FUNCTION_BLOCK FB95
TITLE =Get Operation Mode
//*****************************************************************************
//* maxon motor ag
//* R&D
//* all rights reserved
//*****************************************************************************
//* Summary:  Read operation mode
//*
//* Remarks:
//*
//* Created under: STEP7 REV5.2+SP1
//*****************************************************************************
//* History:
//* 19.05.2004 | INA   first release
//*
//*
//*****************************************************************************
//

AUTHOR:INA
FAMILY:StateMac
NAME:GetOpMod
VERSION:00.01


VAR_INPUT

Read : BOOL //A rising edge start the command

  NodeID : BYTE //Adress of the maxon device

END_VAR
VAR_OUTPUT
  Done : BOOL //Data valid flag is TRUE if data were available

  Err : BOOL //Error flag is TRUE if an Error has occured, see ErrNo for more details

  ErrNo : DINT //Contains detailed error information

  Mode : BYTE //Operation Mode

END_VAR
VAR
  xEdgeMerker : BOOL //Edge Merker

  xEdgeFlag : BOOL //Edge Flag

  xStep : INT
END_VAR

BEGIN

NETWORK
TITLE = Activate the service function
//

// SDO Read "Get Operation Mode"

       U    #Read
       FP   #xEdgeFlag                   // recognize a positiv edge of the Read signal
       =    #xEdgeMerker                 // and set the xEdgeMerker for one cycle to true

       L    #xStep
       L    0
       ==I
       U    #xEdgeMerker
       SPB  nstp                         // iStep = 1 -> fnc1

       L    #xStep                       // jump list
       SPL  List
       SPA  rdef
       SPA  fnc1
       SPA  fncE
List  :SPA  rdef

rdef  :NOP  0
       R    #Done                        // reset Done
       R    #Err                         // reset Error
       L    0
       T    #xStep                       // iStep = 0
       SPA  end

fnc1  :NOP  0
       CALL FC1
         NodeID:=#NodeID
         Index:=DW#16#00006061
         SubIndex:=DW#16#00000000
         RET_VAL:=#Done
         Err:=#Err
         ErrNo:=#ErrNo

       L    DB219.DBB10
       T    #Mode

       L    1
       U    #Err
       SPB  fncE

       SPA  nstp                         // iStep = 1 -> fnc2

fncE  :NOP  0
       L    0
       T    #xStep
       SPA  end

nstp  :NOP  0
       L    #xStep
       INC            1
       T    #xStep

end   :NOP  0
END_FUNCTION_BLOCK
